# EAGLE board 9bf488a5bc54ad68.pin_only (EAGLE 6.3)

Size 22.86 x 25.4 mm. Coordinates in mm from the lower left corner, seen from the top.
Outline: 0,22.86 0,2.54 arc90 2.54,0 20.32,0 arc90 22.86,2.54 22.86,22.86 arc90 20.32,25.4 2.54,25.4 arc90 0,22.86
Copper layers (1*16): Top 0.035mm / dielectric 1.5mm / Bottom 0.035mm
Design rules "adafruit *": minimum track width 8mil, minimum drill 16mil, track to track 8mil, track to pad 8mil, pad to pad 8mil, via to via 8mil, smd to smd 8mil, copper to edge 10mil, drill to drill 8mil, minimum pad ring 10mil, minimum via ring 8mil, stop-mask expansion 4mil, vias tented up to drill 20mil, thermal gap 10mil

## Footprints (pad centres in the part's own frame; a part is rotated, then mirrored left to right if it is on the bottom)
C0805K = smd 1.3 x 1.6: 1 -1,0; 2 1,0
FIDUCIAL_1MM = smd 1 x 1: 1 0,0
SO14 = smd 0.6 x 2.2: 1 -3.81,-2.6; 2 -2.54,-2.6; 3 -1.27,-2.6; 4 0,-2.6; 5 1.27,-2.6; 6 2.54,-2.6; 7 3.81,-2.6; 8 3.81,2.6; 9 2.54,2.6; 10 1.27,2.6; 11 0,2.6; 12 -1.27,2.6; 13 -2.54,2.6; 14 -3.81,2.6
1X06-CLEANBIG = drill 1.016 pad 1.778 octagon: 1 -6.35,0; 2 -3.81,0; 3 -1.27,0; 4 1.27,0; 5 3.81,0; 6 6.35,0
CHIP-LED0805 = smd 1.2 x 1.2: A 0,-1.05; C 0,1.05
R0805 = smd 1.3 x 1.5: 1 -0.95,0; 2 0.95,0
MOUNTINGHOLE_2.5_PLATED = drill 2.5 pad 3.2: P$1 0,0

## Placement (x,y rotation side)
C1  0.1uF  [C0805K]  7.11,6.1 180 top
FID1  FIDUCIAL""  [FIDUCIAL_1MM]  17.65,20.83 0 top
FID2  FIDUCIAL""  [FIDUCIAL_1MM]  11.05,4.06 0 top
IC1  AT42QT1070-SSU  [SO14]  10.92,13.34 90 top
JP1  [1X06-CLEANBIG]  21.59,12.57 90 top
JP3  [1X06-CLEANBIG]  1.27,12.57 270 top
LED1  [CHIP-LED0805]  17.65,8.76 270 top
LED2  [CHIP-LED0805]  17.65,11.3 270 top
LED3  [CHIP-LED0805]  17.65,13.84 270 top
LED4  [CHIP-LED0805]  17.65,16.38 270 top
LED5  [CHIP-LED0805]  17.65,18.92 270 top
R1  10K  [R0805]  4.7,8.76 0 top
R2  10K  [R0805]  4.7,11.3 0 top
R3  10K  [R0805]  4.7,13.84 0 top
R4  10K  [R0805]  4.7,16.26 0 top
R5  10K  [R0805]  4.7,18.92 0 top
R6  470  [R0805]  15.88,6.22 0 top
R7  470  [R0805]  12.83,6.86 270 top
R8  470  [R0805]  10.29,6.86 270 top
R9  470  [R0805]  9.78,18.92 180 top
R10  470  [R0805]  13.84,19.3 180 top
U$1  MOUNTINGHOLE2.5  [MOUNTINGHOLE_2.5_PLATED]  2.54,22.86 0 top
U$2  MOUNTINGHOLE2.5  [MOUNTINGHOLE_2.5_PLATED]  20.32,22.86 0 top
U$3  MOUNTINGHOLE2.5  [MOUNTINGHOLE_2.5_PLATED]  2.54,2.54 0 top
U$4  MOUNTINGHOLE2.5  [MOUNTINGHOLE_2.5_PLATED]  20.32,2.54 0 top
U$6  [ADAFRUIT_5MM]  14.48,0.89 0 bottom

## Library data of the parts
C1 R1-R10 = rcl
FID1 FID2 U$1-U$4 U$6 = microbuilder
IC1 JP1 JP3 = adafruit
LED1-LED5 = led

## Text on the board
tPlace: AT42QT1070 | Standalone | 4 | 4 | 3 | 3 | 2 | 2 | 1 | 1 | 0 | 0 | Gnd | VDD | Input | Output | 5 Cap. Keys | Ch0 is guard key
bPlace: 5 Key Capacitive | Touch Sensors | Only one key is | detected at a time | 6x6mm min pads | VDD: 1.8-5.5VDC

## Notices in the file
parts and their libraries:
microbuilder: This work is placed in the public domain, and may be freely used for commercial and non-commercial work with the following conditions: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
